{attribute 'qualified_only'}
VAR_GLOBAL
//Tolerance
	PRESSURE_WARNING:BOOL;
	PRESSURE_ALARM:BOOL;
	
	MFC1_WARNING:BOOL;
	MFC1_Alarm:BOOL;
	
	MFC2_WARNING:BOOL;
	MFC2_Alarm:BOOL;
	
	MFC3_WARNING:BOOL;
	MFC3_Alarm:BOOL;
	
	MFC4_WARNING:BOOL;
	MFC4_Alarm:BOOL;
	
	MFC5_WARNING:BOOL;
	MFC5_Alarm:BOOL;
	
	MFC6_WARNING:BOOL;
	MFC6_Alarm:BOOL;
	
	MFC7_WARNING:BOOL;
	MFC7_Alarm:BOOL;
	
	MFC8_WARNING:BOOL;
	MFC8_Alarm:BOOL;
	
	MFC9_WARNING:BOOL;
	MFC9_Alarm:BOOL;
	
	WALL_TEMP_WARNING:BOOL;
	WALL_TEMP_Alarm:BOOL;
		
	LID_TEMP_WARNING:BOOL;
	LID_TEMP_Alarm:BOOL;
	
	STAGE_EDGE_TEMP_WARNING:BOOL;
	STAGE_EDGE_TEMP_Alarm:BOOL;
	
	STAGE_CENTER_TEMP_WARNING: BOOL;
	STAGE_CENTER_TEMP_ALARM: BOOL;
	
//INTERLOCK
	STATUS_PrepareTransfer:BOOL;
	STATUS_TransferWafer:BOOL;
	STATUS_OpenGasValve:BOOL;
	STATUS_CloseGasValve:BOOL;
	STATUS_OpenCloseSlitValve:BOOL;
	
	AV1_EN	:BOOL;//	MFC1前气动阀(N2-1)	使能
	AV2_EN	:BOOL;//	MFC1前气动阀(N2-3)	使能
	AV3_EN	:BOOL;//	MFC1后气动阀	使能
	AV4_EN	:BOOL;//	MFC2前气动阀(N2-1)	使能
	AV5_EN	:BOOL;//	MFC2前气动阀(NH3)	使能
	AV6_EN	:BOOL;//	MFC2后气动阀	使能
	AV7_EN	:BOOL;//	MFC3前气动阀(N2-1)	使能
	AV8_EN	:BOOL;//	MFC3前气动阀(NH3)	使能
	AV9_EN	:BOOL;//	MFC3后气动阀	使能
	AV10_EN	:BOOL;//	N2-1 总进气阀	使能
	AV11_EN	:BOOL;//	MFC1,2,3 BYPASS阀(N2-1)	使能
	AV12_EN	:BOOL;//	N2-2 总进气阀	使能
	AV13_EN	:BOOL;//	MFC5,6,7 BYPASS阀(N2-2)	使能
	AV14_EN	:BOOL;//	MFC5前气动阀(N2-2)	使能
	AV15_EN	:BOOL;//	MFC5前气动阀(HF)	使能
	AV16_EN	:BOOL;//	MFC5后气动阀	使能
	AV17_EN	:BOOL;//	OF前气动阀(N2-2)	使能
	AV18_EN	:BOOL;//	OF前气动阀(HF)	使能
	AV19_EN	:BOOL;//	OF后气动阀	使能
	AV20_EN	:BOOL;//	MFC6前气动阀(N2-2)	使能
	AV21_EN	:BOOL;//	MFC6前气动阀(Ar)	使能
	AV22_EN	:BOOL;//	MFC6后气动阀	使能
	AV23_EN	:BOOL;//	MFC7前气动阀(N2-2)	使能
	AV24_EN	:BOOL;//	MFC7前气动阀(Ar)	使能
	AV25_EN	:BOOL;//	MFC7后气动阀	使能
	AV26_EN	:BOOL;//	Chamber总进气阀(NH3,N2)	使能
	AV27_EN	:BOOL;//	Chamber总进气阀(HF,Ar)	使能
	AV101_EN:BOOL;//	Dry Pump至Chamber	使能
	AV102_EN:BOOL;//	Dry Pump至TMP	使能
	AV103_EN:BOOL;//	TMP N2 Purge	使能
	AV104_EN:BOOL;//	VG103压力计前置保护阀	使能
	AV105_EN:BOOL;//	BA01压力计前置保护阀	使能
	AV106_EN:BOOL;//	酸排阀	使能
	APC_EN	:BOOL;//	APC Open	使能

	AV1_EN_Bypass	:BOOL;//	MFC1前气动阀(N2-1)	使能Bypass
	AV2_EN_Bypass	:BOOL;//	MFC1前气动阀(N2-3)	使能Bypass
	AV3_EN_Bypass	:BOOL;//	MFC1后气动阀	使能Bypass
	AV4_EN_Bypass	:BOOL;//	MFC2前气动阀(N2-1)	使能Bypass
	AV5_EN_Bypass	:BOOL;//	MFC2前气动阀(NH3)	使能Bypass
	AV6_EN_Bypass	:BOOL;//	MFC2后气动阀	使能Bypass
	AV7_EN_Bypass	:BOOL;//	MFC3前气动阀(N2-1)	使能Bypass
	AV8_EN_Bypass	:BOOL;//	MFC3前气动阀(NH3)	使能Bypass
	AV9_EN_Bypass	:BOOL;//	MFC3后气动阀	使能Bypass
	AV10_EN_Bypass	:BOOL;//	N2-1 总进气阀	使能Bypass
	AV11_EN_Bypass	:BOOL;//	MFC1,2,3 BYPASS阀(N2-1)	使能Bypass
	AV12_EN_Bypass	:BOOL;//	N2-2 总进气阀	使能Bypass
	AV13_EN_Bypass	:BOOL;//	MFC5,6,7 BYPASS阀(N2-2)	使能Bypass
	AV14_EN_Bypass	:BOOL;//	MFC5前气动阀(N2-2)	使能Bypass
	AV15_EN_Bypass	:BOOL;//	MFC5前气动阀(HF)	使能Bypass
	AV16_EN_Bypass	:BOOL;//	MFC5后气动阀	使能Bypass
	AV17_EN_Bypass	:BOOL;//	OF前气动阀(N2-2)	使能Bypass
	AV18_EN_Bypass	:BOOL;//	OF前气动阀(HF)	使能Bypass
	AV19_EN_Bypass	:BOOL;//	OF后气动阀	使能Bypass
	AV20_EN_Bypass	:BOOL;//	MFC6前气动阀(N2-2)	使能Bypass
	AV21_EN_Bypass	:BOOL;//	MFC6前气动阀(Ar)	使能Bypass
	AV22_EN_Bypass	:BOOL;//	MFC6后气动阀	使能Bypass
	AV23_EN_Bypass	:BOOL;//	MFC7前气动阀(N2-2)	使能Bypass
	AV24_EN_Bypass	:BOOL;//	MFC7前气动阀(Ar)	使能Bypass
	AV25_EN_Bypass	:BOOL;//	MFC7后气动阀	使能Bypass
	AV26_EN_Bypass	:BOOL;//	Chamber总进气阀(NH3,N2)	使能Bypass
	AV27_EN_Bypass	:BOOL;//	Chamber总进气阀(HF,Ar)	使能Bypass
	AV101_EN_Bypass	:BOOL;//	Dry Pump至Chamber	使能Bypass
	AV102_EN_Bypass	:BOOL;//	Dry Pump至TMP	使能Bypass
	AV103_EN_Bypass	:BOOL;//	TMP N2 Purge	使能Bypass
	AV104_EN_Bypass	:BOOL;//	VG103压力计前置保护阀	使能Bypass
	AV105_EN_Bypass	:BOOL;//	BA01压力计前置保护阀	使能Bypass
	AV106_EN_Bypass	:BOOL;//	酸排阀	使能Bypass
	APC_EN_Bypass	:BOOL;//	APC Open	使能Bypass

	HTR_APC_EN,
	HTR_CHAMBER_EN,
	HTR_FORLINE_EN,
	HTR_GAS_BOX_EN,
	HTR_GATE_VALVE_EN,
	HTR_LID_EN:BOOL;
	
	HTR_APC_EN_Bypass,
	HTR_CHAMBER_EN_Bypass,
	HTR_FORLINE_EN_Bypass,
	HTR_GAS_BOX_EN_Bypass,
	HTR_GATE_VALVE_EN_Bypass,
	HTR_LID_EN_Bypass:BOOL;
	
//PROCESS
	Process_RUN: BOOL;
	Process_Stop: BOOL;
	
//SPLC
	Lid_Temp_OT_Bypass,
	Chamber_Temp_OT_Bypass,
	APC_Temp_OT_Bypass,
	Gate_Valve_Temp_OT_Bypass,
	Gas_Line_Temp_OT_Bypass	,
	Stage_Temp_OT_Bypass	,
	TMP_ALARM_Bypass	,
	PS1_ALM_Bypass,
	PS2_ALM_Bypass,
	SPLC_manual_ErrorAck	:BOOL;	
	SPLC_TO_PLC	AT	%I*	:SPLC_TO_PLC;
	PLC_TO_SPLC	AT	%Q*	:PLC_TO_SPLC;
	
(*	
	Lid_Temp_OK,
	Chamber_Temp_OK,
	APC_Temp_OK,
	Gate_Valve_Temp_OK,
	Gas_Line_Temp_OK	,
	TMP_Interlock_OK	,
	PS1_Interlock_OK	,
	PS2_Interlock_OK	AT	%Q*	:BOOL;	
	
	EV1_EN,
	EV2_EN,
	EV3_EN,
	EV4_EN,
	HTR_APC_EN,
	HTR_CHAMBER_EN,
	HTR_FORLINE_EN,
	HTR_GAS_BOX,
	HTR_GATE_VALVE,
	HTR_LID,
	PROCESS_EN,
	TMP_PW_EN,
	TRANSFER_EN,
	VALVE_ACID_EXHAUST_OPEN_EN,
	VALVE_CM_OPEN_EN,
	VALVE_DRY_PUMP_OPEN_EN,
	VALVE_TMP_BACK_OPEN_EN,
	VALVE_APC_OPEN_EN,
	WAFER_MOVING_IN_EN	AT	%I*	:BOOL;
	
	SPLC_ErrorAcknowledgement,
	SPLC_manual_ErrorAck,
	SPLC_Restart,
	SPLC_Run	AT	%Q*	:BOOL;			
	SPLC_Com_err,
	SPLC_FB_Err AT	%I*	:BOOL;
	*)
	
	
END_VAR
